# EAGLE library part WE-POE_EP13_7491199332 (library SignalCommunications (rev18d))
Power over Ethernet Transformer Characteristics Flyback transformer designed for PoE PDs Input voltage: 36 V to 57 V Switching frequencies: 200–500 kHz Operating temperature: –40 ºC to +125 ºC Insulation test voltage: 1.5 kVAC/1 min Different output powers and voltages available Applications Suitable for PoE IC’s like LTC4267, TPS 23750, TPS 23770, LM5070, LM 5071, LM 5072 Details see: http://katalog.we-online.de/en/pbs/WE-PoE? Updated by Dan Xu 2014-07-08 2014 (C) Wurth Elektronik
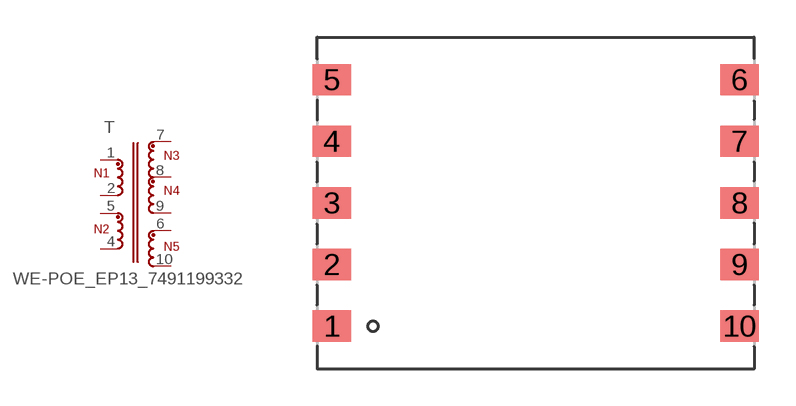
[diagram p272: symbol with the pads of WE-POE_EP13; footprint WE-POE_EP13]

Designator prefix T

## WE-POE_EP13_7491199332  [WE-POE_EP13]
1  1  pas
2  2  pas
4  4  pas
5  3  pas
6  8  pas
7  5  pas
8  6  pas
9  7  pas
10  9  pas

## Footprint WE-POE_EP13 (pad centres in mm)
smd 1.55 x 1.27: 1 -8.275,-5; 2 -8.275,-2.5; 3 -8.275,0; 4 -8.275,2.5; 5 -8.275,5; 6 8.275,5; 7 8.275,2.5; 8 8.275,0; 9 8.275,-2.5; 10 8.275,-5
